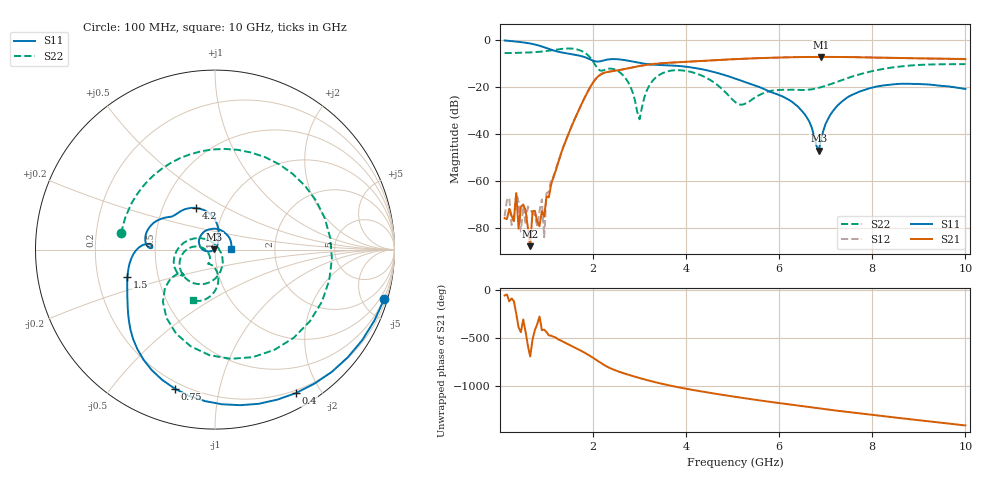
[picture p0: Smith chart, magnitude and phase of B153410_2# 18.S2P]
!  2-Port S-parameters saved by WinCal
! VAR MeasName=S-Parameters (CALIBRATED_DATA) read from VNA (N5245A)
! VAR MeasDate=2016-12-23 10:00:16
! VAR NAME=B153410_2# 18
! VAR FILENAME=B153410_2# 18.S2P
! VAR DATE=2016-12-23 10:00:16
! VAR PHYS_PORTS=1,2
# Hz S DB R 50
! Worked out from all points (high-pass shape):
!   199 points, 100 MHz to 10 GHz, reference 50 ohm
!   highest |S21| = -7.14 dB at 6.9 GHz (marker M1); lowest = -87.8 dB at 650 MHz (marker M2)
!   |S21| within 3 dB of the highest: 3.311 GHz to end of sweep
!   lowest |S11| = -47.1 dB at 6.85 GHz (marker M3), VSWR 1.01, Z = 49.6 + j0.203 ohm
!   |S11| at or under -10 dB: 3.09 GHz to end of sweep
!   |S22| runs from -33.7 to -3.6 dB; largest |S21 - S12| = 0.0033
!   S11 on the Smith chart (normalised r, x): 100 MHz: 0.44, -7.00; 400 MHz: 0.17, -1.70; 750 MHz: 0.17, -0.74; 1.5 GHz: 0.33, -0.13; 4.2 GHz: 0.74, +0.36; 10 GHz: 1.20, +0.01
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1e8  -0.15 -16.2  -75.87 -52.7  -75.11 -179.8  -5.51 170.2
3e8  -0.52 -46.3  -77.14 -113.2  -75.08 122.6  -5.49 150.3
3.5e8  -0.63 -53.4  -65.15 115.0  -65.09 -67.4  -5.48 145.1
4e8  -0.74 -60.6  -80.31 -27.2  -68.80 -96.3  -5.45 139.8
4.5e8  -0.87 -67.4  -70.97 -77.5  -81.50 125.1  -5.42 134.4
6.5e8  -1.45 -93.8  -87.77 26.9  -72.30 82.9  -5.27 111.1
7.5e8  -1.87 -106.2  -72.73 -57.0  -74.51 -57.0  -5.15 98.3
9e8  -2.72 -123.0  -72.90 -56.6  -67.84 -60.0  -4.88 77.0
9.5e8  -3.06 -128.0  -75.24 -51.0  -83.96 -12.5  -4.77 69.4
1e9  -3.41 -132.5  -66.61 -76.2  -65.19 -75.5  -4.64 61.4
1.5e9  -5.84 -162.9  -38.66 147.0  -38.64 147.2  -3.58 -37.1
1.75e9  -6.83 -176.8  -27.41 85.0  -27.39 85.4  -4.60 -93.0
2.65e9  -8.43 158.5  -12.44 -147.3  -12.44 -147.5  -15.10 166.8
3e9  -9.70 146.9  -11.02 161.2  -11.05 161.0  -33.72 22.2
3.4e9  -10.58 139.6  -9.98 110.1  -9.99 109.9  -15.14 -95.1
4.2e9  -11.92 114.1  -9.05 31.4  -9.06 31.3  -14.10 -166.5
5.05e9  -16.37 87.1  -8.10 -35.6  -8.13 -35.6  -26.30 -173.7
6.7e9  -37.34 64.8  -7.16 -147.5  -7.18 -147.4  -20.97 -100.3
6.85e9  -47.06 152.5  -7.15 -156.9  -7.16 -157.0  -20.32 -94.3
6.9e9  -42.21 -172.1  -7.14 -160.1  -7.15 -160.0  -20.06 -92.3
8.35e9  -19.06 135.0  -7.56 114.4  -7.57 114.4  -11.88 -94.3
1e10  -20.80 3.5  -8.10 23.8  -8.13 24.0  -10.23 -113.3
